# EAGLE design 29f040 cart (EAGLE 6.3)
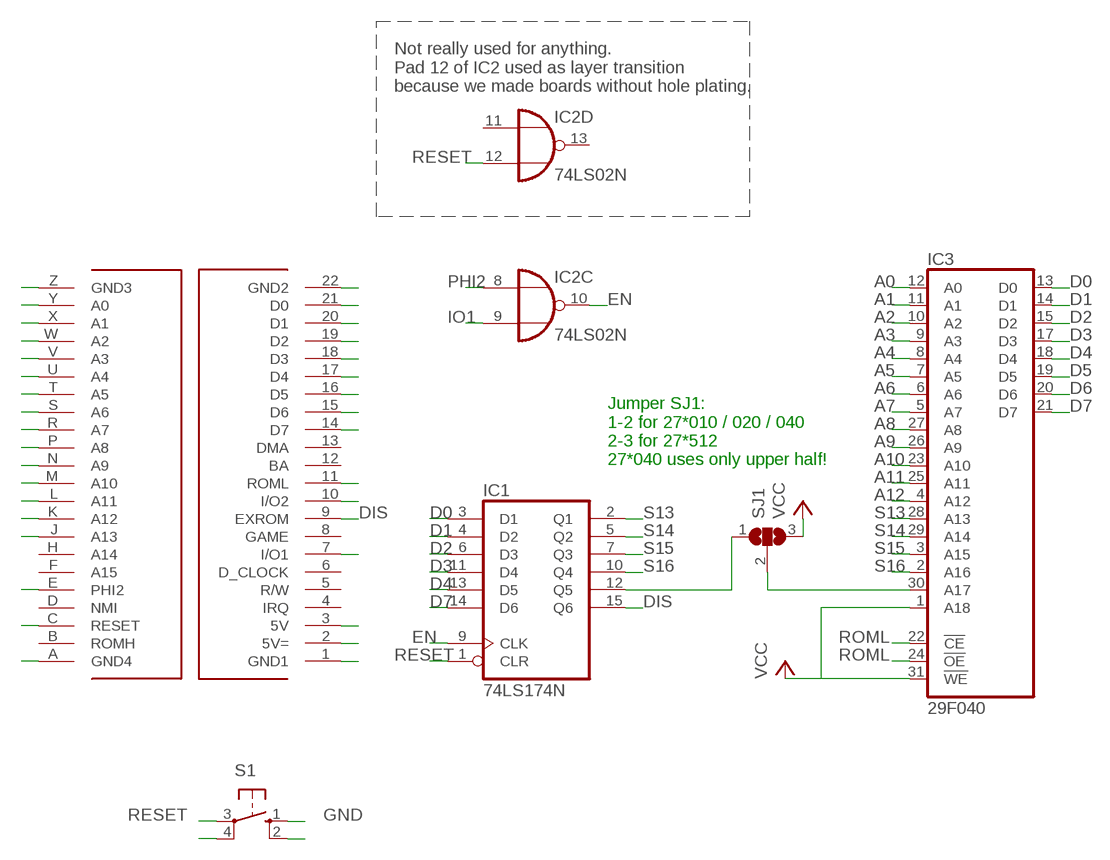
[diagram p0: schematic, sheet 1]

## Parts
IC1  74LS174N  [DIL16]
IC2  74LS02N  [DIL14]
IC3  29F040  AM29F040N  [DIL32-6]
S1  10-XX  [B3F-10XX]
SJ1  SJ2W  [SJ_2]
U$1  C64_EXPANSION__CARTRIDGE  [C64_EXPANSION__CARTRIDGE]

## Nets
A0: IC3.12(A0) U$1.Y(A0)
A1: IC3.11(A1) U$1.X(A1)
A2: IC3.10(A2) U$1.W(A2)
A3: IC3.9(A3) U$1.V(A3)
A4: IC3.8(A4) U$1.U(A4)
A5: IC3.7(A5) U$1.T(A5)
A6: IC3.6(A6) U$1.S(A6)
A7: IC3.5(A7) U$1.R(A7)
A8: IC3.27(A8) U$1.P(A8)
A9: IC3.26(A9) U$1.N(A9)
A10: IC3.23(A10) U$1.M(A10)
A11: IC3.25(A11) U$1.L(A11)
A12: IC3.4(A12) U$1.K(A12)
A13: U$1.J(A13)
D0: IC1.3(D1) IC3.13(D0) U$1.21(D0)
D1: IC1.4(D2) IC3.14(D1) U$1.20(D1)
D2: IC1.6(D3) IC3.15(D2) U$1.19(D2)
D3: IC1.11(D4) IC3.17(D3) U$1.18(D3)
D4: IC1.13(D5) IC3.18(D4) U$1.17(D4)
D5: IC3.19(D5) U$1.16(D5)
D6: IC3.20(D6) U$1.15(D6)
D7: IC1.14(D6) IC3.21(D7) U$1.14(D7)
DIS: IC1.15(Q6) U$1.9(EXROM)
EN: IC1.9(CLK) IC2.10(C:O)
GND: S1.1(S) S1.2(S1) U$1.1(GND1) U$1.22(GND2) U$1.A(GND4) U$1.Z(GND3)
IO1: IC2.9(C:I1) U$1.7(I/O1)
IO2: U$1.10(I/O2)
N$4: IC3.30(A17) SJ1.2
N$5: IC1.12(Q5) SJ1.1
PHI2: IC2.8(C:I0) U$1.E(PHI2)
RESET: IC1.1(CLR) IC2.12(D:I1) S1.3(P) S1.4(P1) U$1.C(RESET)
ROML: IC3.22(!CE) IC3.24(!OE) U$1.11(ROML)
S13: IC1.2(Q1) IC3.28(A13)
S14: IC1.5(Q2) IC3.29(A14)
S15: IC1.7(Q3) IC3.3(A15)
S16: IC1.10(Q4) IC3.2(A16)
VCC: IC3.1(A18) IC3.31(!WE) SJ1.3 U$1.2(5V=) U$1.3(5V)
Unconnected: IC2.1(A:O) IC2.2(A:I0) IC2.3(A:I1) IC2.4(B:O) IC2.5(B:I0) IC2.6(B:I1) IC2.11(D:I0) IC2.13(D:O) U$1.4(IRQ) U$1.5(R/W) U$1.6(D_CLOCK) U$1.8(GAME) U$1.12(BA) U$1.13(DMA) U$1.B(ROMH) U$1.D(NMI) U$1.F(A15) U$1.H(A14)

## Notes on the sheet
- Not really used for anything.
  Pad 12 of IC2 used as layer transition
  because we made boards without hole plating.
- Jumper SJ1:
  1-2 for 27*010 / 020 / 040
  2-3 for 27*512
  27*040 uses only upper half!

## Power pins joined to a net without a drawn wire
GND: IC1.8(GND) IC2.7(P:GND) IC3.16(GND)
VCC: IC1.16(VCC) IC2.14(P:VCC) IC3.32(VCC)

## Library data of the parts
IC1 = 74xx-eu:74*174: Hex D type FLIP FLOP, clear
IC2 = 74xx-eu:74*02: Quad 2-input NOR gate
IC3 = 0RB_Memory:AM29F040: 4-Megabit FLASH MEMORY (512 K x 8 bit) 5 V-only
S1 = switch-omron:10-XX: OMRON SWITCH; MPN: B3F-1000; OC_FARNELL: 176432; OC_NEWARK: 36M3542
SJ1 = jumper:SJ2W: SMD solder JUMPER
U$1 = 64kb_cart:C64_EXPANSION__CARTRIDGE

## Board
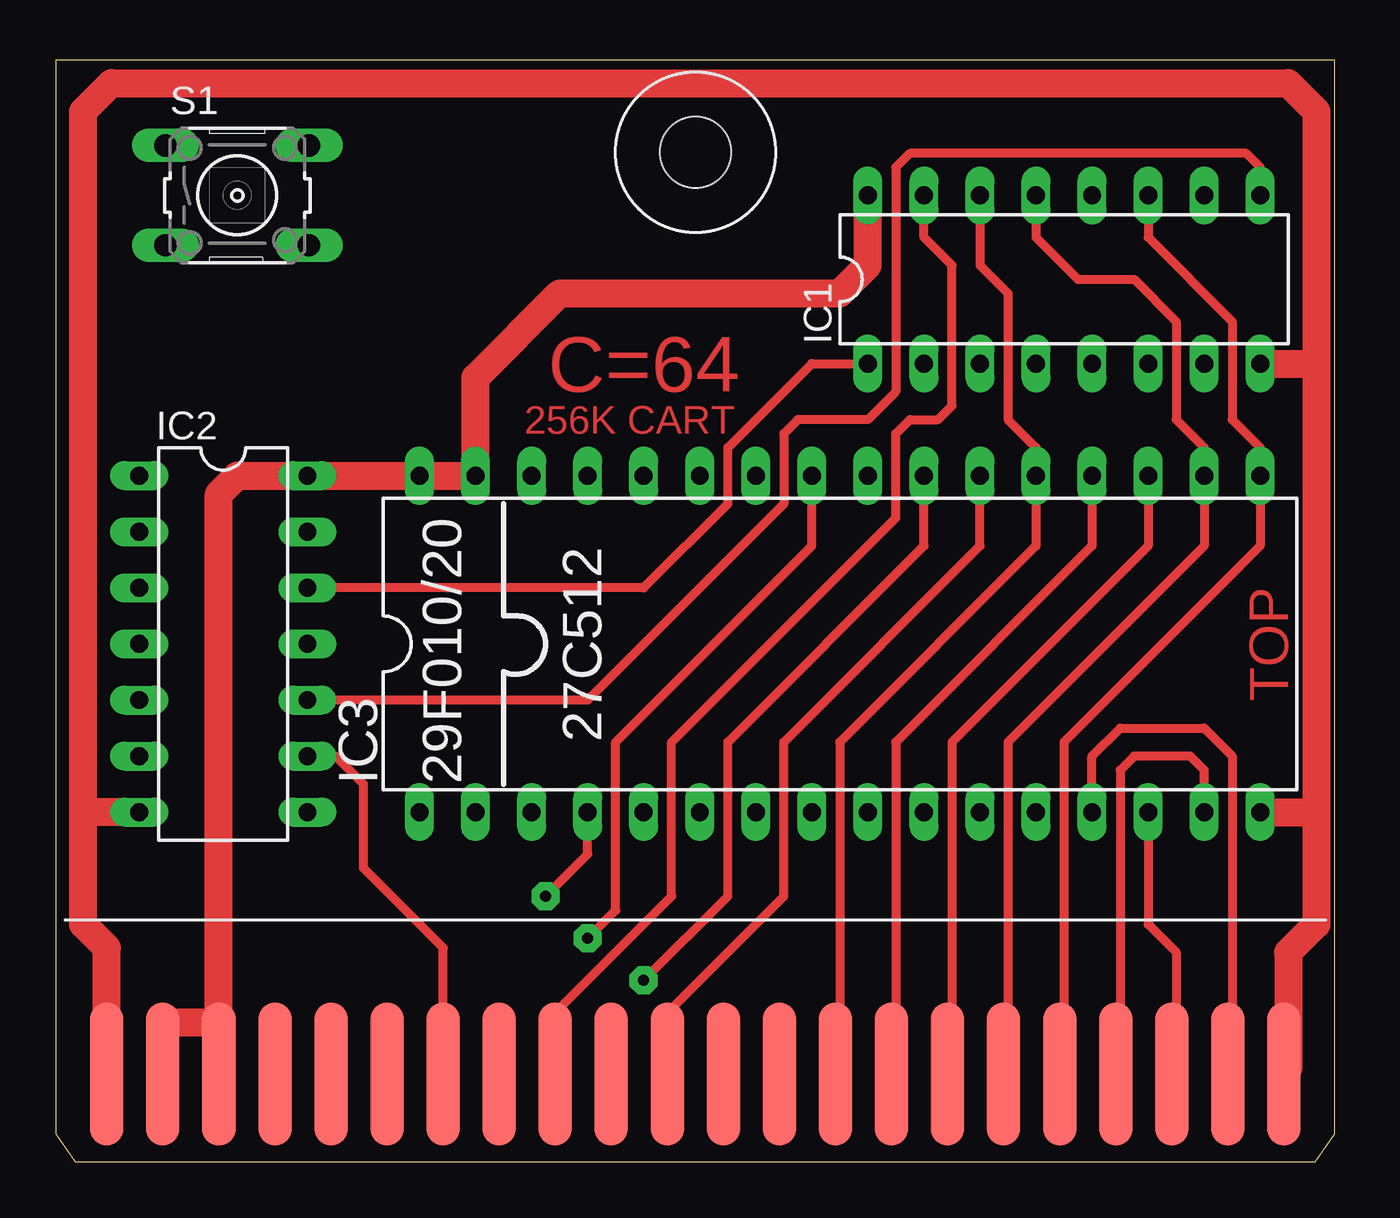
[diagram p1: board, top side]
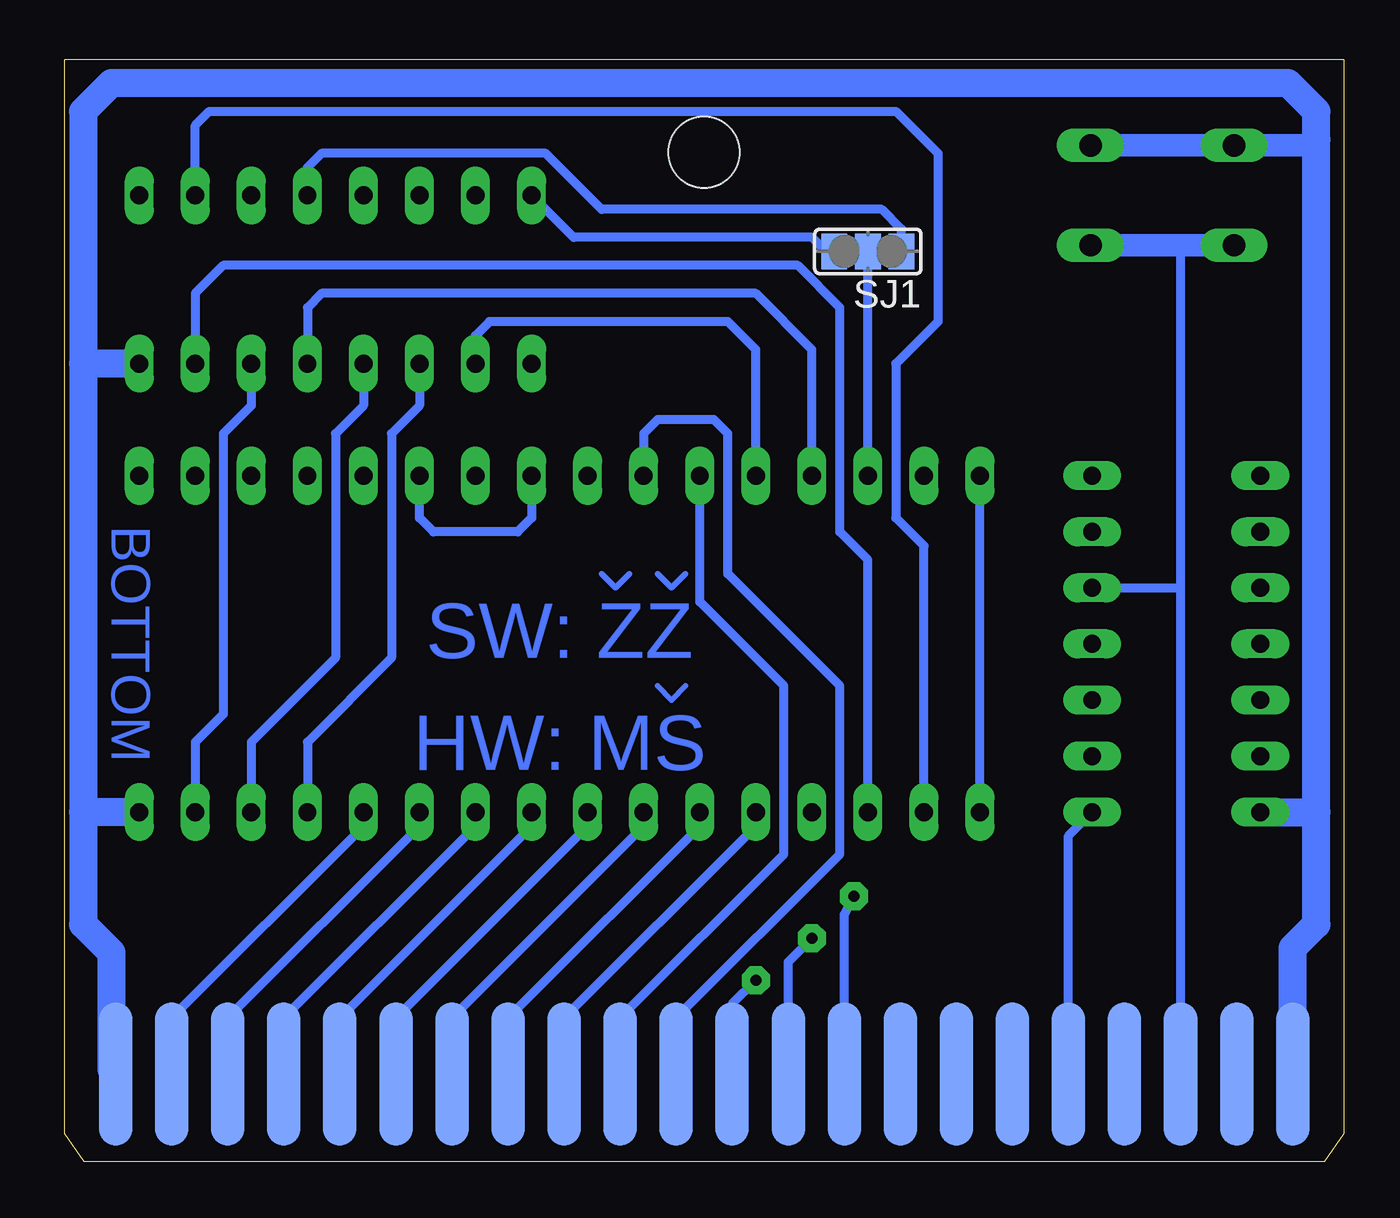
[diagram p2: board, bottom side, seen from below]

Size 57.98 x 49.93 mm. Coordinates in mm from the lower left corner, seen from the top.
Copper layers (1*16): Top 0.035mm / dielectric 1.5mm / Bottom 0.035mm
Design rules "elecrow_eagle_rule_v1.1": minimum track width 6mil, minimum drill 12mil, track to track 6mil, track to pad 6mil, pad to pad 6mil, via to via 6mil, smd to smd 0mil, copper to edge 10mil, drill to drill 10mil, minimum pad ring 10mil, minimum via ring 6mil, stop-mask expansion 2mil, vias tented up to drill 100mil, thermal gap 10mil

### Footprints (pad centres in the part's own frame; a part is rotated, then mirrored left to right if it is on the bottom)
DIL16 = drill 0.813 long: 1 -8.89,-3.81; 2 -6.35,-3.81; 3 -3.81,-3.81; 4 -1.27,-3.81; 5 1.27,-3.81; 6 3.81,-3.81; 7 6.35,-3.81; 8 8.89,-3.81; 9 8.89,3.81; 10 6.35,3.81; 11 3.81,3.81; 12 1.27,3.81; 13 -1.27,3.81; 14 -3.81,3.81; 15 -6.35,3.81; 16 -8.89,3.81
DIL14 = drill 0.813 long: 1 -7.62,-3.81; 2 -5.08,-3.81; 3 -2.54,-3.81; 4 0,-3.81; 5 2.54,-3.81; 6 5.08,-3.81; 7 7.62,-3.81; 8 7.62,3.81; 9 5.08,3.81; 10 2.54,3.81; 11 0,3.81; 12 -2.54,3.81; 13 -5.08,3.81; 14 -7.62,3.81
DIL32-6 = drill 0.813 long: 1 -19.05,-7.62; 2 -16.51,-7.62; 3 -13.97,-7.62; 4 -11.43,-7.62; 5 -8.89,-7.62; 6 -6.35,-7.62; 7 -3.81,-7.62; 8 -1.27,-7.62; 9 1.27,-7.62; 10 3.81,-7.62; 11 6.35,-7.62; 12 8.89,-7.62; 13 11.43,-7.62; 14 13.97,-7.62; 15 16.51,-7.62; 16 19.05,-7.62; 17 19.05,7.62; 18 16.51,7.62; 19 13.97,7.62; 20 11.43,7.62; 21 8.89,7.62; 22 6.35,7.62; 23 3.81,7.62; 24 1.27,7.62; 25 -1.27,7.62; 26 -3.81,7.62; 27 -6.35,7.62; 28 -8.89,7.62; 29 -11.43,7.62; 30 -13.97,7.62; 31 -16.51,7.62; 32 -19.05,7.62
B3F-10XX = drill 1.016 long: 1 -3.251,2.261; 2 3.251,2.261; 3 -3.251,-2.261; 4 3.251,-2.261
SJ_2 = smd 1.168 x 1.6: 1 -1.524,0; 2 0,0; 3 1.524,0
C64_EXPANSION__CARTRIDGE = smd 1.524 x 6.477: 1 2.34,4.01; 2 4.88,4.01; 3 7.42,4.01; 4 9.96,4.01; 5 12.5,4.01; 6 15.04,4.01; 7 17.58,4.01; 8 20.12,4.01; 9 22.66,4.01; 10 25.2,4.01; 11 27.74,4.01; 12 30.28,4.01; 13 32.82,4.01; 14 35.36,4.01; 15 37.9,4.01; 16 40.44,4.01; 17 42.98,4.01; 18 45.52,4.01; 19 48.06,4.01; 20 50.6,4.01; 21 53.14,4.01; 22 55.68,4.01 | smd 1.524 x 6.477 bottom: A 2.34,4.01; B 4.88,4.01; C 7.42,4.01; D 9.96,4.01; E 12.5,4.01; F 15.04,4.01; H 17.58,4.01; J 20.12,4.01; K 22.66,4.01; L 25.2,4.01; M 27.74,4.01; N 30.28,4.01; P 32.82,4.01; R 35.36,4.01; S 37.9,4.01; T 40.44,4.01; U 42.98,4.01; V 45.52,4.01; W 48.06,4.01; X 50.6,4.01; Y 53.14,4.01; Z 55.68,4.01 | hole 3.2: 29.01,45.761

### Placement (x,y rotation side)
IC1  45.7,39.96 0 top
IC2  7.6,23.45 270 top
IC3  35.54,23.45 0 top
S1  8.23,43.77 0 top
SJ1  21.57,41.23 180 bottom
U$1  -0.02,-0.04 0 top

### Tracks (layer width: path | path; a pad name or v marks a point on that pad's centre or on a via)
A0
  Bottom 0.406: IC3.12 44.43,15.2 53.32,6.31 53.32,4.17
  Bottom 0.61: 53.32,4.17 U$1.Y
A1
  Bottom 0.406: IC3.11 41.89,15.2 50.78,6.31 50.78,4.17
  Bottom 0.61: 50.78,4.17 U$1.X
A2
  Bottom 0.406: IC3.10 39.35,15.2 48.24,6.31 48.24,4.17
  Bottom 0.61: 48.24,4.17 U$1.W
A3
  Bottom 0.406: IC3.9 36.81,15.2 45.06,6.94 45.06,4.4
  Bottom 0.61: 45.06,4.4 U$1.V
A4
  Bottom 0.406: IC3.8 34.27,15.2 42.52,6.94 42.52,4.4
  Bottom 0.61: 42.52,4.4 U$1.U
A5
  Bottom 0.406: IC3.7 31.73,15.2 40.62,6.31 40.62,4.17
  Bottom 0.61: 40.62,4.17 U$1.T
A6
  Bottom 0.406: IC3.6 29.19,15.2 37.44,6.94 37.44,4.4
  Bottom 0.61: 37.44,4.4 U$1.S
A7
  Bottom 0.406: IC3.5 26.65,15.2 35.54,6.31 35.54,4.17
  Bottom 0.61: 35.54,4.17 U$1.R
A8
  Bottom 0.406: U$1.P 32.8,6.51 25.38,13.93 25.38,21.55 29.19,25.36 IC3.27
A9
  Bottom 0.406: U$1.N 30.26,6.51 22.84,13.93 22.84,21.55 27.92,26.63 27.92,32.98 28.55,33.61 31.09,33.61 31.73,32.98 IC3.26
A10  (via drill 0.5 pad 1.27)
  Top 0.406: v26.65,8.21 30.46,12.02 30.46,19.01 39.35,27.9 IC3.23
  Bottom 0.406: U$1.M 27.72,7.14 v26.65,8.21
A11  (via drill 0.5 pad 1.27)
  Top 0.406: v24.11,10.12 25.38,11.39 25.38,19.01 34.27,27.9 IC3.25
  Bottom 0.406: U$1.L 25.18,9.05 v24.11,10.12
A12  (via drill 0.5 pad 1.27)
  Top 0.406: v22.2,12.02 24.11,13.93 IC3.4
  Bottom 0.406: U$1.K 22.64,11.19 v22.2,12.02
D0
  Top 0.406: IC3.13 46.97,18.37 48.24,19.64 52.05,19.64 53.32,18.37 53.32,4.17
  Top 0.61: 53.32,4.17 U$1.21
  Bottom 0.406: IC1.3 41.89,34.25 43.16,32.98 43.16,22.82 46.97,19.01 IC3.13
D1
  Top 0.406: IC3.14 49.51,10.75 50.78,9.48 50.78,4.17
  Top 0.61: 50.78,4.17 U$1.20
  Bottom 0.406: IC1.4 44.43,34.25 45.7,32.98 45.7,22.82 49.51,19.01 IC3.14
D2
  Top 0.406: IC3.15 52.05,17.74 51.41,18.37 48.87,18.37 48.24,17.74 48.24,4.17
  Top 0.61: 48.24,4.17 U$1.19
  Bottom 0.406: IC1.6 49.51,34.25 50.78,32.98 50.78,20.28 52.05,19.01 IC3.15
D3
  Top 0.406: 45.7,4.17 45.7,19.01 54.59,27.9 IC3.17 54.59,32.34 53.32,33.61 53.32,38.06 49.51,41.87 IC1.11
  Top 0.61: 45.7,4.17 U$1.18
D4
  Top 0.406: 43.16,4.17 43.16,19.01 52.05,27.9 IC3.18 52.05,32.34 50.78,33.61 50.78,38.06 48.87,39.96 46.33,39.96 44.43,41.87 IC1.13
  Top 0.61: 43.16,4.17 U$1.17
D5
  Top 0.406: IC3.19 49.51,27.9 40.62,19.01 40.62,4.17
  Top 0.61: 40.62,4.17 U$1.16
D6
  Top 0.406: IC3.20 46.97,27.9 38.08,19.01 38.08,4.17
  Top 0.61: 38.08,4.17 U$1.15
D7
  Top 0.406: 35.54,4.17 35.54,19.01 44.43,27.9 IC3.21 44.43,32.34 43.16,33.61 43.16,39.33 41.89,40.6 IC1.14
  Top 0.61: 35.54,4.17 U$1.14
DIS
  Top 0.406: U$1.9 22.64,6.74 27.92,12.02 27.92,19.01 38.08,29.17 38.08,32.98 38.71,33.61 39.98,33.61 40.62,34.25 40.62,40.6 39.35,41.87 IC1.15
EN
  Top 0.406: IC1.9 54.59,45.04 53.95,45.68 38.71,45.68 38.08,45.04 38.08,34.88 36.81,33.61 33.63,33.61 33,32.98 33,29.8 24.11,20.91 IC2.10
GND
  Top 1.27: U$1.A 2.32,9.68 1.25,10.75 1.25,15.83 | 1.25,15.83 1.25,47.58 2.52,48.85 55.86,48.85 57.13,47.58 57.13,36.15 | 57.13,36.15 57.13,15.83 | 57.13,15.83 57.13,10.75 55.86,9.48 55.86,4.17 U$1.22 | IC3.16 57.13,15.83 | IC1.8 57.13,36.15 | IC2.7 1.25,15.83
  Bottom 1.016: S1.2 S1.1 1.53,46.03 1.25,46.31
  Bottom 1.27: U$1.A 2.32,9.68 1.25,10.75 1.25,15.83 | 1.25,15.83 1.25,46.31 1.25,47.58 2.52,48.85 55.86,48.85 57.13,47.58 57.13,36.15 | 57.13,36.15 57.13,15.83 | 57.13,15.83 57.13,10.75 55.86,9.48 55.86,4.17 U$1.22 | IC2.7 1.25,15.83 | IC3.16 57.13,15.83 | IC1.8 57.13,36.15
IO1
  Top 0.406: U$1.7 17.56,9.68 13.95,13.29 13.95,17.1 12.68,18.37 IC2.9
N$1
  Bottom 0.254: 29.82,26.63 30.46,25.99 31.09,26.63
N$2
  Bottom 0.254: 32.36,26.63 33,25.99 33.63,26.63
N$3
  Bottom 0.254: 29.82,21.55 30.46,20.91 31.09,21.55
N$4
  Bottom 0.406: IC3.30 SJ1.2
N$5
  Bottom 0.406: SJ1.1 20.04,42.25 20.93,43.14 33.63,43.14 36.17,45.68 46.33,45.68 46.97,45.04 IC1.12
PHI2
  Bottom 0.406: U$1.E 12.48,14.76 IC2.8
RESET
  Top 0.406: IC2.12 26.65,25.99 30.46,29.8 30.46,32.34 34.27,36.15 IC1.1
  Bottom 0.406: U$1.C 7.4,25.99 | 7.4,25.99 7.4,41.08 6.96,41.51 | IC2.12 7.4,25.99
  Bottom 1.016: S1.4 6.96,41.51 S1.3
ROML
  Top 0.406: U$1.11 27.72,6.74 33,12.02 33,19.01 41.89,27.9 IC3.22
  Bottom 0.406: IC3.24 36.81,29.17 37.44,28.53 41.25,28.53 41.89,29.17 IC3.22
S13
  Bottom 0.406: IC3.28 26.65,36.79 27.92,38.06 38.71,38.06 39.35,37.42 IC1.2
S14
  Bottom 0.406: IC3.29 24.11,36.79 26.65,39.33 46.33,39.33 46.97,38.69 IC1.5
S15
  Bottom 0.406: IC3.3 21.57,27.26 22.84,28.53 22.84,38.69 24.74,40.6 50.78,40.6 52.05,39.33 IC1.7
S16
  Bottom 0.406: IC3.2 19.03,27.9 20.3,29.17 20.3,36.15 18.39,38.06 18.39,45.68 20.3,47.58 51.41,47.58 52.05,46.95 IC1.10
VCC
  Top 0.406: U$1.3 7.4,6.31 | 4.86,6.11 5.06,6.31
  Top 1.27: IC1.16 36.81,40.6 35.54,39.33 22.84,39.33 19.03,35.52 IC3.31 IC3.32 IC2.14 8.23,31.07 7.4,30.24 7.4,6.31 5.06,6.31 | U$1.2 4.86,6.11
  Bottom 0.406: IC3.1 IC3.32 | IC1.16 34.9,41.87 24.11,41.87 23.47,41.23 SJ1.3

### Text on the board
Top: C=64 | 256K CART | TOP
Bottom: BOTTOM | SW: ZZ / HW: MS
tNames: 27C512 | 29F010/20
bValues: 3 2 1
